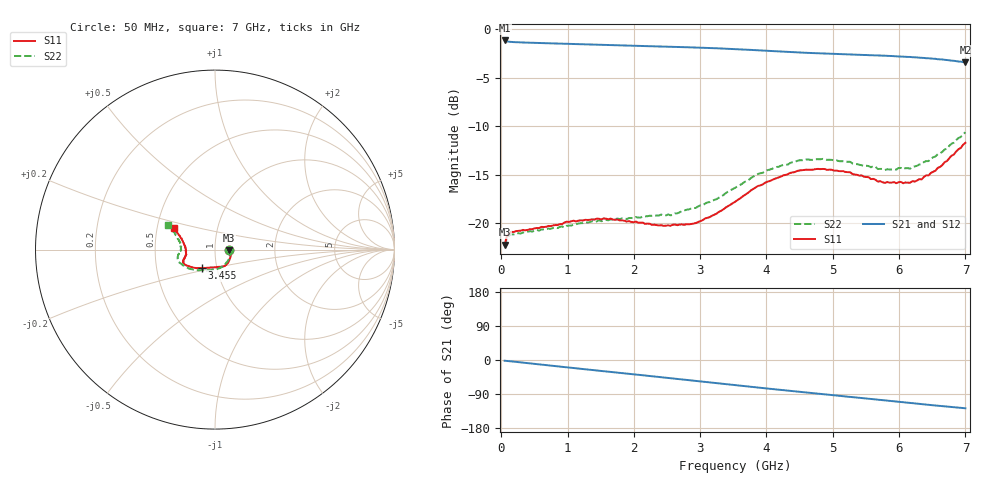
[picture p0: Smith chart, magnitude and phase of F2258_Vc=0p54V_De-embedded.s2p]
! Integrated Device Technology
! Corporate Headquarters
! 6024 Silver Creek Valley Road
! San Jose, CA 95138  USA
! Phone:  1-408-284-8200
! Toll Free:  1-800-223-1366
! Webpage:  http://www.idt.com/
! Timing and RF Division
! 515 Groton Road, Suite 102
! Westford, MA 01886-6024
! Device:  F2258
! Description: Voltage Variable RF Attenuator
! Frequency:  50.0 -  6000.00 MHz
! Package:  3x3 mm Thin QFN Plastic Package: 16 pin
! Ports:  2 RF, 2 DC
!  Pin  1  = NC
!  Pin  2  = NC
!  Pin  3  = RF2  = Port 2
!  Pin  4  = GND
!  Pin  5  = Vdd
!  Pin  6  = NC
!  Pin  7  = VCTRL
!  Pin  8  = NC
!  Pin  9  = GND
!  Pin 10  = RF1  = Port 1
!  Pin 11  = NC
!  Pin 12  = NC
!  Pin 13  = NC
!  Pin 14  = NC
!  Pin 15  = NC
!  Pin 16  = NC
! Vcntrl:  0.540 Volts
! Vdd:  +3.300 Volts
! Current:  1.104 mA
! Data:  The device was measured on a the F2258 evaluation board which has
!  individual transmission lines to the RF pins.  Data was collected
!  using a calibrated network analyzer.  The evaluation board was
!  de-embedded using a TRL calibration technique.
!  The reference plane is the edge of the package pin.
! Misc:  SN 10
!  Action Tracker AT0285
! Date Measured:  2014-12-10
! Date:  2016-01-13  MJV
! Note:
!  Integrated Device Technology supplies this data as a sample of measured
!  data at the package pin for this product.  Your particular data for this
!  product may vary.
!  Data was taken at 25 degrees C.
!  Integrated Device Technology reserves the right to change this data at anytime.
!Freq_(GHz)  S11M_(dB)  S11P_(deg)  S21M_(dB)  S21P_(deg)  S12M_(dB)  S12P_(deg)  S22M_(dB)  S22P_(deg)
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# GHz S dB R 50
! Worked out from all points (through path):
!   201 points, 50 MHz to 7 GHz, reference 50 ohm
!   highest |S21| = -1.16 dB at 50 MHz (marker M1); lowest = -3.4 dB at 7 GHz (marker M2)
!   group delay of S21, straight-line fit = 50.5 ps
!   lowest |S11| = -22.2 dB at 50 MHz (marker M3), VSWR 1.17, Z = 58.4 - j0.463 ohm
!   |S11| at or under -10 dB: start of sweep to end of sweep
!   |S22| runs from -22.3 to -10.6 dB; largest |S21 - S12| = 0.00046
!   S11 on the Smith chart (normalised r, x): 50 MHz: 1.17, -0.01; 3.455 GHz: 0.85, -0.18; 7 GHz: 0.61, +0.16
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0.05  -22.19 -2.9  -1.16 -2.0  -1.16 -2.0  -22.34 -3.0
0.08475  -21.30 -4.7  -1.25 -2.5  -1.25 -2.5  -21.47 -4.8
0.15425  -20.86 -7.3  -1.31 -3.7  -1.31 -3.7  -21.12 -8.3
0.71025  -20.25 -30.5  -1.45 -14.1  -1.44 -14.1  -20.52 -34.4
1.2315  -19.70 -50.0  -1.56 -23.9  -1.56 -23.9  -19.96 -57.7
1.6485  -19.50 -60.8  -1.64 -31.5  -1.64 -31.5  -19.59 -70.8
2.37825  -20.21 -79.6  -1.77 -44.8  -1.77 -44.8  -19.18 -89.5
2.552  -20.23 -85.2  -1.80 -48.0  -1.81 -48.0  -19.16 -94.8
2.93425  -19.96 -101.6  -1.88 -55.1  -1.89 -55.1  -18.40 -108.5
3.247  -18.99 -115.4  -1.96 -61.0  -1.96 -61.0  -17.49 -120.9
3.4555  -18.07 -124.9  -2.02 -64.9  -2.03 -64.9  -16.58 -128.7
3.525  -17.77 -127.4  -2.04 -66.2  -2.05 -66.2  -16.33 -131.8
4.0115  -15.70 -143.4  -2.22 -75.3  -2.22 -75.3  -14.51 -148.0
4.46325  -14.59 -152.8  -2.38 -83.4  -2.39 -83.4  -13.55 -159.5
4.7065  -14.45 -156.2  -2.46 -87.7  -2.46 -87.7  -13.44 -163.9
5.2625  -14.72 -162.8  -2.61 -97.4  -2.61 -97.4  -13.65 -172.3
5.6795  -15.69 -168.8  -2.70 -104.6  -2.70 -104.6  -14.39 -178.1
5.85325  -15.79 -173.0  -2.75 -107.7  -2.75 -107.7  -14.43 177.3
6.166  -15.80 178.9  -2.85 -113.3  -2.86 -113.3  -14.36 171.1
6.33975  -15.47 172.1  -2.94 -116.4  -2.94 -116.4  -13.87 166.6
6.722  -13.57 158.7  -3.17 -123.1  -3.17 -123.0  -12.30 157.3
7  -11.69 152.2  -3.42 -127.4  -3.42 -127.4  -10.61 152.2
